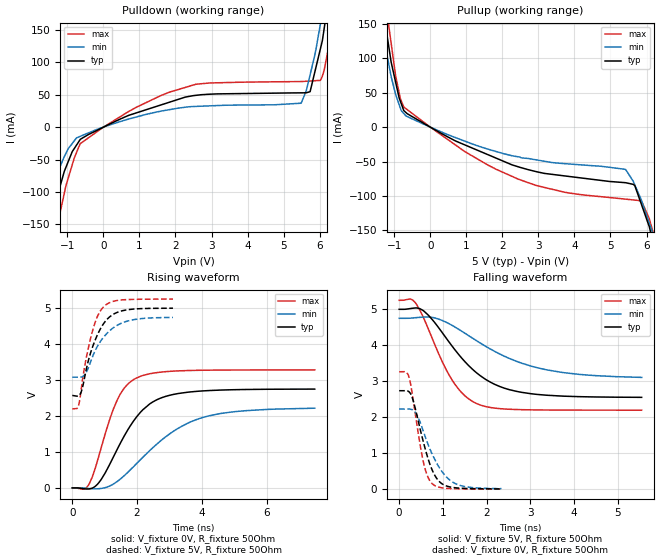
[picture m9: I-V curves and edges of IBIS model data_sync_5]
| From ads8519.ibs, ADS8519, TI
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|   data_sync_5 Model
[Model]   data_sync_5
Model_type   Output
Polarity   Non-Inverting
Vmeas = 2.5
Vref = 2.5
Cref = 5pF
Rref = 50
|   typ   min   max
|   (nom PVT)   (Fast PVT)   (slow PVT)
| C_comp by Frequency method (F=29Mhz)
|Average
|C_comp   1.005e-11   9.006e-12   1.136e-11
|ON state : BUFFER OUTPUT TURNED HIGH
|C_comp   1.005e-11   9.006e-12   1.136e-11
|OFF state: BUFFER OUTPUT TURNED LOW
|C_comp   9.192e-12   8.384e-12   1.013e-11
| C_comp by LC Tank method (L=1nH)
| Resonant frequency (Hz)  1.86e9   1.94e9   1.79e9
C_comp   7.329e-12   6.758e-12   7.914e-12
| Where nom  PVT is Nominal Process,  5V,  32C
|   Fast PVT is Strong Process,   5.25V,  -40C
|   Slow PVT is Weak Process,   4.75V,  92C
[Voltage Range]   5   4.75   5.25
|Ambient Temperature   25   85   -40
|Junction Temperature
[Temperature Range]   32   92   -40
[Pullup Reference]   5   4.75   5.25
[Pulldown Reference]   0   0   0
[Power Clamp Reference]   5   4.75   5.25
[GND Clamp Reference]   0   0   0
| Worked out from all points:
|   slope of the pulldown table from 0 to 0.75 V, typ, clamps not added: 39.4 ohm
|   slope of the pullup table from 0 to 0.75 V, typ, clamps not added: 35.3 ohm
|   falling waveform, V_fixture 5V, R_fixture 50Ohm: 20-80 % time 1.1ns typ, 1.59ns min, 740ps max; typ from 5 V to 2.56 V
|   rising waveform, V_fixture 0V, R_fixture 50Ohm: 20-80 % time 1.12ns typ, 1.78ns min, 748ps max; typ from 0 V to 2.75 V
|   rising waveform, V_fixture 5V, R_fixture 50Ohm: 20-80 % time 548ps typ, 680ps min, 434ps max; typ from 2.57 V to 5 V
|   falling waveform, V_fixture 0V, R_fixture 50Ohm: 20-80 % time 368ps typ, 496ps min, 269ps max; typ from 2.74 V to 0.011 V
[Pulldown]
|   Voltage   I(typ)   I(min)   I(max)
-5V       -999.1mA   -732.8mA   -1.367A
-1.824V   -231.2mA   -154.4mA   -326.8mA
-1.302V   -110.6mA   -73.98mA   -157.2mA
-651mV    -19.66mA   -14.34mA   -26.33mA
693mV     17.98mA    12.38mA    23.87mA
2.567V    49.02mA    31.95mA    66.15mA
5.481V    52.86mA    36.85mA    70.27mA
5.735V    54.71mA    80.74mA    71.12mA
6.016V    119.9mA    157.8mA    72.08mA
6.3V      217.2mA    247.5mA    148mA
6.525V    304.9mA    318.7mA    255.8mA
10V       1.482A     1.326A     1.714A
[Pullup]
|   Voltage   I(typ)   I(min)   I(max)
-5V       1.402A     1.207A     1.7A
-1.969V   419.7mA    345.4mA    514.8mA
-1.306V   170mA      134.2mA    206.5mA
-1.088V   95.36mA    74.09mA    122.9mA
-960.7mV  65.24mA    47.55mA    74.67mA
-735mV    24.04mA    19.84mA    29.49mA
2.452V    -57.87mA   -43.26mA   -75.88mA
5.415V    -80.79mA   -61.41mA   -104.7mA
5.675V    -85.15mA   -84.12mA   -106.1mA
5.859V    -112.5mA   -106.5mA   -107.3mA
6.179V    -166.7mA   -155.2mA   -152.6mA
10V       -1.092A    -847.4mA   -1.401A
[Ramp]
R_load = 50
|   typ   min   max
dV/dt_r   1.64867/1.11428e-09   1.33877/1.80311e-09   1.96697/7.47094e-10
dV/dt_f   1.46989/1.10414e-09   1.00257/1.64301e-09   1.83103/7.39446e-10
[Falling Waveform]
V_fixture = 5V
V_fixture_min = 4.75V
V_fixture_max = 5.25V
R_fixture = 50Ohm
|   Time   V(typ)   V(min)   V(max)
0s        5V         4.75V      5.25V
260ps     5.022V     4.754V     5.284V
370ps     5.037V     4.766V     5.183V
670ps     4.832V     4.787V     4.445V
1.19ns    4.009V     4.567V     3.075V
1.5ns     3.548V     4.337V     2.601V
1.77ns    3.235V     4.126V     2.382V
2.42ns    2.803V     3.688V     2.23V
3.35ns    2.615V     3.324V     2.203V
5.54ns    2.555V     3.108V     2.198V
[Rising Waveform]
V_fixture = 0V
V_fixture_min = 0V
V_fixture_max = 0V
R_fixture = 50Ohm
|   Time   V(typ)   V(min)   V(max)
0s        3.744nV    4.393nV    3.296nV
360ps     -23.54mV   -5.261mV   -33.7mV
510ps     -29.23mV   -17.49mV   89.94mV
900ps     243.4mV    -14.89mV   1.138V
1.39ns    1.076V     179.7mV    2.446V
1.63ns    1.482V     360.6mV    2.801V
1.99ns    1.977V     678.6mV    3.058V
2.71ns    2.489V     1.293V     3.216V
4.03ns    2.696V     1.957V     3.27V
7.49ns    2.746V     2.216V     3.278V
[Rising Waveform]
V_fixture = 5V
V_fixture_min = 4.75V
V_fixture_max = 5.25V
R_fixture = 50Ohm
|   Time   V(typ)   V(min)   V(max)
0s        2.57V      3.078V     2.198V
190ps     2.558V     3.078V     2.277V
300ps     2.738V     3.088V     2.896V
410ps     3.2V       3.179V     3.511V
580ps     3.795V     3.539V     4.207V
750ps     4.2V       3.892V     4.707V
950ps     4.543V     4.169V     5.016V
1.25ns    4.816V     4.438V     5.182V
1.66ns    4.945V     4.625V     5.233V
3.11ns    4.995V     4.74V      5.249V
[Falling Waveform]
V_fixture = 0V
V_fixture_min = 0V
V_fixture_max = 0V
R_fixture = 50Ohm
|   Time   V(typ)   V(min)   V(max)
0s        2.738V     2.23V      3.265V
160ps     2.738V     2.23V      3.255V
230ps     2.704V     2.229V     3.091V
380ps     2.19V      2.119V     2.004V
540ps     1.379V     1.657V     834.5mV
630ps     974.6mV    1.346V     426.3mV
740ps     578.2mV    1.016V     174mV
950ps     180.1mV    542.5mV    47.17mV
1.28ns    43.18mV    161mV      15.98mV
2.34ns    11.09mV    18.41mV    3.928mV
